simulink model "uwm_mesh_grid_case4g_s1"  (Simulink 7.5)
settings: Solver=ode45  StartTime=0.0  StopTime=8.0  RelTol=1e-4
undefined symbols (not defined in the file or in its folder): D1, Delta, dfilt, DiscIntNeverNeededParam
libraries: powerlib x90, powerlib_extras x24, dsparch4 x6
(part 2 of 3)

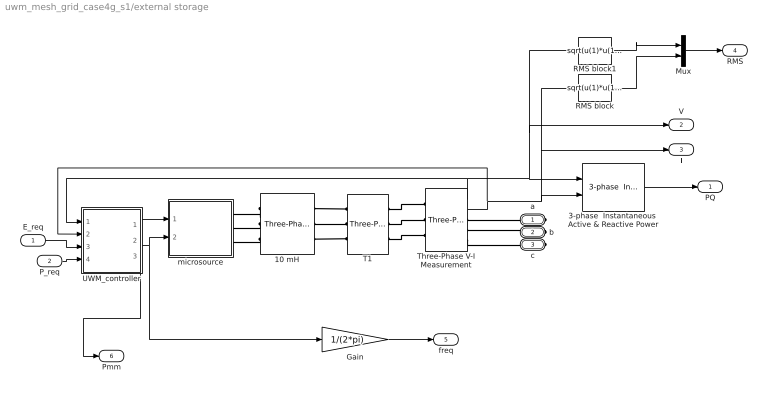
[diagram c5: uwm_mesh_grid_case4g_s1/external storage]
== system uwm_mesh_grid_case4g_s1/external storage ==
  E_req : Inport
  P_req : Inport  Port=2
  10 mH : powerlib/Elements/Three-Phase Series RLC Branch  DialogController=POWERSYS.PowerSysDialog  PhysicalDomain=powersysdomain  SubClassName=unknown  LeftPortType=p1  RightPortType=p1  LConnTagsString=A|B|C  RConnTagsString=A|B|C  BranchType=L  Resistance=.0028  Inductance=5e-3  Capacitance=1e-6  Measurements=None
  3-phase  Instantaneous  Active & Reactive Power : powerlib_extras/Measurements/3-phase  Instantaneous  Active & Reactive Power  DialogController=POWERSYS.PowerSysDialog  SystemSampleTime=-1
  Gain : Gain  Gain=1/(2*pi)  ParameterDataType=fixdt(1, 16)  ParameterScaling=2^0  OutDataType=fixdt(1, 16)  OutScaling=2^0
  Mux : Mux  Inputs=2
  RMS block : Fcn  Expr=sqrt(u(1)*u(1)+u(2)*u(2)+u(3)*u(3))/sqrt(3)
  RMS block1 : Fcn  Expr=sqrt(u(1)*u(1)+u(2)*u(2)+u(3)*u(3))/sqrt(3)
  T1 : powerlib/Elements/Three-Phase Transformer (Two Windings)  DialogController=POWERSYS.PowerSysDialog  SystemSampleTime=-1  Winding1Connection=Delta (D1)  UNITS=SI  NominalPower=[ 45e3 , 60 ]  Winding1=[208 0.02688 0.1075/(2*pi*60)]  Winding2Connection=Yg  Winding2=[208 0.005047 .0201/(2*pi*60)]  SetSaturation=off  Rm=100.e6  Lm=7650.8  Saturation=[0 0;1359.8 0.93633;5.6659e+05 1.186]  Hysteresis=off  DataFile='hysteresis'  SetInitialFlux=off  InitialFluxes=[0.62422 -0.62422 0.54618]  Measurements=None  MoreParameters=off  BreakLoop=off  DataType=on  TransfoNumber=1
  Three-Phase V-I Measurement : powerlib/Measurements/Three-Phase V-I Measurement  DialogController=POWERSYS.PowerSysDialog  SystemSampleTime=-1  VoltageMeasurement=phase-to-ground  SetLabelV=off  LabelV=Vabc  Vpu=off  VpuLL=off  CurrentMeasurement=yes  SetLabelI=off  LabelI=Iabc  Ipu=off  Pbase=100e6  Vbase=500e3  OutputType=Complex  PhasorSimulation=off  PSBequivalent=0
  UWM_controller : Subsystem  mask{Vbase=208, Sbase=15000}
  microsource : Subsystem
  a : PMIOPort  Port=1  Side=Right
  b : PMIOPort  Port=2  Side=Right
  c : PMIOPort  Port=3  Side=Right
  PQ : Outport  OutDataType=fixdt(1, 16)  OutScaling=2^0
  V : Outport  Port=2  OutDataType=fixdt(1, 16)  OutScaling=2^0
  I : Outport  Port=3  OutDataType=fixdt(1, 16)  OutScaling=2^0
  RMS : Outport  Port=4  OutDataType=fixdt(1, 16)  OutScaling=2^0
  freq : Outport  Port=5  OutDataType=fixdt(1, 16)  OutScaling=2^0
  Pmm : Outport  Port=6
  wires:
  E_req/1 -> UWM_controller/3(E_req)
  P_req/1 -> UWM_controller/4(P_req)
  Three-Phase V-I Measurement/1 -> UWM_controller/1(v_meas), 3-phase  Instantaneous  Active & Reactive Power/1, RMS block1/1, V/1
  Three-Phase V-I Measurement/2 -> UWM_controller/2(i_meas), 3-phase  Instantaneous  Active & Reactive Power/2, RMS block/1, I/1
  UWM_controller/1(Vpk) -> microsource/1(Vpk)
  UWM_controller/2(w) -> microsource/2(w), Gain/1
  Gain/1 -> freq/1
  3-phase  Instantaneous  Active & Reactive Power/1 -> PQ/1
  RMS block1/1 -> Mux/1
  RMS block/1 -> Mux/2
  Mux/1 -> RMS/1
  UWM_controller/3(Pmm) -> Pmm/1
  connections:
  b/RConn1 -- Three-Phase V-I Measurement/RConn2
  Three-Phase V-I Measurement/RConn3 -- c/RConn1
  10 mH/LConn2 -- microsource/RConn2
  10 mH/LConn1 -- microsource/RConn1
  10 mH/LConn3 -- microsource/RConn3
  T1/LConn1 -- 10 mH/RConn1
  T1/LConn2 -- 10 mH/RConn2
  T1/LConn3 -- 10 mH/RConn3
  T1/RConn1 -- Three-Phase V-I Measurement/LConn1
  T1/RConn2 -- Three-Phase V-I Measurement/LConn2
  T1/RConn3 -- Three-Phase V-I Measurement/LConn3
  a/RConn1 -- Three-Phase V-I Measurement/RConn1

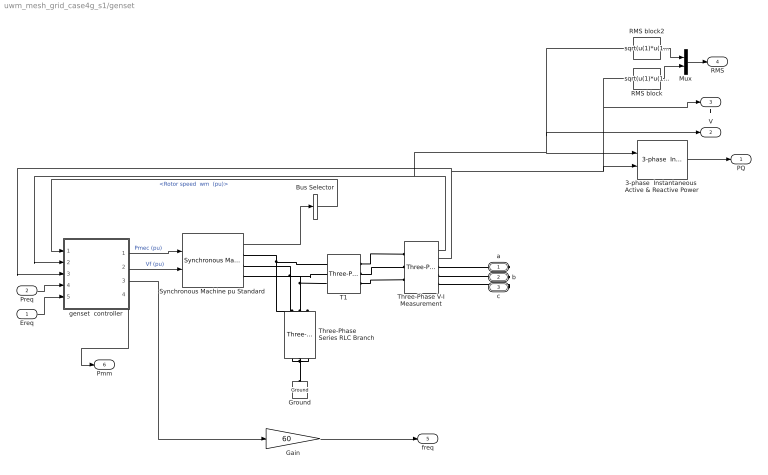
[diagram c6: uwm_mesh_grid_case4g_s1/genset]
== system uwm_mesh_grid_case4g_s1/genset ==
  Ereq : Inport  OutDataType=fixdt(1, 16)  OutScaling=2^0
  Preq : Inport  Port=2  OutDataType=fixdt(1, 16)  OutScaling=2^0
  3-phase  Instantaneous  Active & Reactive Power : powerlib_extras/Measurements/3-phase  Instantaneous  Active & Reactive Power  DialogController=POWERSYS.PowerSysDialog  SystemSampleTime=-1
  Bus Selector : BusSelector  OutputSignals="Mechanical.Rotor speed  wm  (pu)"
  Gain : Gain  Gain=60  ParameterDataType=fixdt(1, 16)  ParameterScaling=2^0  OutDataType=fixdt(1, 16)  OutScaling=2^0
  Ground : powerlib/Elements/Ground  DialogController=POWERSYS.PowerSysDialog  PhysicalDomain=powersysdomain  SubClassName=unknown  LeftPortType=p1  RightPortType=p1  LConnTagsString=a
  Mux : Mux  Inputs=2
  RMS block : Fcn  Expr=sqrt(u(1)*u(1)+u(2)*u(2)+u(3)*u(3))/sqrt(3)
  RMS block2 : Fcn  Expr=sqrt(u(1)*u(1)+u(2)*u(2)+u(3)*u(3))/sqrt(3)
  Synchronous Machine pu Standard : powerlib/Machines/Synchronous Machine pu Standard  DialogController=POWERSYS.PowerSysDialog  SystemSampleTime=-1  PresetModel=No  MechanicalLoad=Mechanical power Pm  ShowDetailedParameters=on  RotorType=Salient-pole  NominalParameters="[ 12500  208   60]"  Reactances1=[ 1.81, 0.3, 0.23, 1.76, 0.65, 0.25, 0.15 ]  Reactances2="[ 1.204, 0.125, 0.056, 0.533,  0.051,  0.037 ]"  dAxisTimeConstants=Short-circuit  qAxisTimeConstants=Short-circuit  TimeConstants1="[ 4.4849  0.0681  0.1  ]"  TimeConstants2=[ 8.0, 0.03, 1.0, 0.07 ]  TimeConstants3="[  .35523  0.00015  0.067  ]"  TimeConstants4=[ 8.0, 0.03, 0.3371, 0.0295 ]  TimeConstants5=[ 1.01, 0.053, 0.1 ]  TimeConstants6=[ 1.3201, 0.023, 1.0, 0.07 ]  TimeConstants7=[0.35523 0.00015 0.0067]  TimeConstants8=[ 1.3201, 0.0231, 0.3371, 0.0295 ]  StatorResistance=0.0217  Mechanical=[ .19 0 2 ]  PolePairs=2  InitialConditions="[ 0  0  0  0  0  0  0  0  1 ]"  SetSaturation=off  Saturation=[0.6404,0.7127,0.8441,0.9214,0.9956,1.082,1.19,1.316,1.457;0.7,0.7698,0.8872,0.9466,0.9969,1.046,1.1,1.151,1.201]  Units=per unit standard parameters  LoadFlowParameters=[1 0 0 0 0]  TsPowergui=0  TsBlock=-1  IterativeModel=Forward Euler
  T1 : powerlib/Elements/Three-Phase Transformer (Two Windings)  DialogController=POWERSYS.PowerSysDialog  SystemSampleTime=-1  Winding1Connection=Delta (D1)  UNITS=SI  NominalPower=[ 45e3 , 60 ]  Winding1=[208 .02688 .10752/(2*pi*60)]  Winding2Connection=Yg  Winding2=[208 .005047 .201899/(2*pi*60)]  SetSaturation=off  Rm=1e+08  Lm=7650.8  Saturation=[0 0;1359.8 0.93633;5.6659e+05 1.186]  Hysteresis=off  DataFile='hysteresis'  SetInitialFlux=off  InitialFluxes=[0.62422 -0.62422 0.54618]  Measurements=None  MoreParameters=off  BreakLoop=off  DataType=on  TransfoNumber=1
  Three-Phase Series RLC Branch : powerlib/Elements/Three-Phase Series RLC Branch  DialogController=POWERSYS.PowerSysDialog  PhysicalDomain=powersysdomain  SubClassName=unknown  LeftPortType=p1  RightPortType=p1  LConnTagsString=A|B|C  RConnTagsString=A|B|C  BranchType=C  Resistance=1  Inductance=1e-3  Capacitance=1.e-4  Measurements=None
  Three-Phase V-I Measurement : powerlib/Measurements/Three-Phase V-I Measurement  DialogController=POWERSYS.PowerSysDialog  SystemSampleTime=-1  VoltageMeasurement=phase-to-ground  SetLabelV=off  LabelV=Vabc  Vpu=off  VpuLL=off  CurrentMeasurement=yes  SetLabelI=off  LabelI=Iabc  Ipu=off  Pbase=100e6  Vbase=500e3  OutputType=Complex  PhasorSimulation=off  PSBequivalent=0
  genset  controller : Subsystem  mask{Vbase=208, Sbase=12500}
  a : PMIOPort  Port=1  Side=Right
  b : PMIOPort  Port=2  Side=Right
  c : PMIOPort  Port=3  Side=Right
  PQ : Outport  OutDataType=fixdt(1, 16)  OutScaling=2^0
  V : Outport  Port=2  OutDataType=fixdt(1, 16)  OutScaling=2^0
  I : Outport  Port=3  OutDataType=fixdt(1, 16)  OutScaling=2^0
  RMS : Outport  Port=4  OutDataType=fixdt(1, 16)  OutScaling=2^0
  freq : Outport  Port=5  OutDataType=fixdt(1, 16)  OutScaling=2^0
  Pmm : Outport  Port=6
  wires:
  genset  controller/1(Pmech) -> Synchronous Machine pu Standard/1  "Pmec (pu)"
  genset  controller/2(Vf) -> Synchronous Machine pu Standard/2  "Vf (pu)"
  Synchronous Machine pu Standard/1 -> Bus Selector/1
  Bus Selector/1 -> genset  controller/1(wr)  "<Rotor speed  wm  (pu)>"
  Three-Phase V-I Measurement/1 -> genset  controller/2(Vabc), 3-phase  Instantaneous  Active & Reactive Power/1, RMS block2/1, V/1
  Three-Phase V-I Measurement/2 -> genset  controller/3(Iabc), 3-phase  Instantaneous  Active & Reactive Power/2, RMS block/1, I/1
  Preq/1 -> genset  controller/4(Preq)
  Ereq/1 -> genset  controller/5(Ereq1)
  genset  controller/3(w) -> Gain/1
  Gain/1 -> freq/1
  3-phase  Instantaneous  Active & Reactive Power/1 -> PQ/1
  RMS block2/1 -> Mux/1
  RMS block/1 -> Mux/2
  Mux/1 -> RMS/1
  genset  controller/4(Pmm) -> Pmm/1
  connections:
  Three-Phase Series RLC Branch/RConn2 -- Three-Phase Series RLC Branch/RConn1 -- Ground/LConn1 -- Three-Phase Series RLC Branch/RConn3
  Synchronous Machine pu Standard/RConn1 -- T1/LConn1 -- Three-Phase Series RLC Branch/LConn1
  Synchronous Machine pu Standard/RConn2 -- T1/LConn2 -- Three-Phase Series RLC Branch/LConn2
  Synchronous Machine pu Standard/RConn3 -- T1/LConn3 -- Three-Phase Series RLC Branch/LConn3
  T1/RConn2 -- Three-Phase V-I Measurement/LConn2
  T1/RConn1 -- Three-Phase V-I Measurement/LConn1
  T1/RConn3 -- Three-Phase V-I Measurement/LConn3
  Three-Phase V-I Measurement/RConn1 -- a/RConn1
  b/RConn1 -- Three-Phase V-I Measurement/RConn2
  c/RConn1 -- Three-Phase V-I Measurement/RConn3

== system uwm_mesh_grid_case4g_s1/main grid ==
  4.16kV 2500kVA : powerlib/Electrical Sources/Three-Phase Source  DialogController=POWERSYS.PowerSysDialog  SystemSampleTime=-1  Voltage=4160  PhaseAngle=0  Frequency=60  InternalConnection=Yg  SpecifyImpedance=on  Resistance=25^2/1000/10  Inductance=25^2/1000/377  ShortCircuitLevel=1200e6  BaseVoltage=4160  XRratio=100
  PC1 : Subsystem  mask{R=.093400, L=.025500, C=2894.3}
  T1 : powerlib/Elements/Three-Phase Transformer (Two Windings)  DialogController=POWERSYS.PowerSysDialog  SystemSampleTime=-1  Winding1Connection=Delta (D1)  UNITS=SI  NominalPower=[ 2500e3 , 60 ]  Winding1=[4160 .04706 .1882/(2*pi*60)]  Winding2Connection=Yg  Winding2=[480 .000627 .0025068/(2*pi*60)]  SetSaturation=off  Rm=1.e6  Lm=1.e6  Saturation=[0 0;589.26 2.1608;2.4552e+05 2.737]  Hysteresis=off  DataFile='hysteresis'  SetInitialFlux=off  InitialFluxes=[1.4405 -1.4405 1.2604]  Measurements=None  MoreParameters=off  BreakLoop=off  DataType=on  TransfoNumber=1
  T2 : powerlib/Elements/Three-Phase Transformer (Two Windings)  DialogController=POWERSYS.PowerSysDialog  SystemSampleTime=-1  Winding1Connection=Delta (D1)  UNITS=SI  NominalPower=[ 75e3 , 60 ]  Winding1=[480 .0169 .0676/(2*pi*60)]  Winding2Connection=Yg  Winding2=[208 .0003 .0127/(2*pi*60)]  SetSaturation=off  Rm=1.e6  Lm=1.e6  Saturation=[0 0;589.26 2.1608;2.4552e+05 2.737]  Hysteresis=off  DataFile='hysteresis'  SetInitialFlux=off  InitialFluxes=[1.4405 -1.4405 1.2604]  Measurements=None  MoreParameters=off  BreakLoop=off  DataType=on  TransfoNumber=1
  A : PMIOPort  Port=1  Side=Right
  B : PMIOPort  Port=2  Side=Right
  C : PMIOPort  Port=3  Side=Right
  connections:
  A/RConn1 -- T2/RConn1
  B/RConn1 -- T2/RConn2
  C/RConn1 -- T2/RConn3
  T1/RConn1 -- PC1/LConn1
  T1/RConn2 -- PC1/LConn2
  T1/RConn3 -- PC1/LConn3
  PC1/RConn1 -- T2/LConn1
  PC1/RConn2 -- T2/LConn2
  PC1/RConn3 -- T2/LConn3
  4.16kV 2500kVA/RConn2 -- T1/LConn2
  4.16kV 2500kVA/RConn1 -- T1/LConn1
  4.16kV 2500kVA/RConn3 -- T1/LConn3

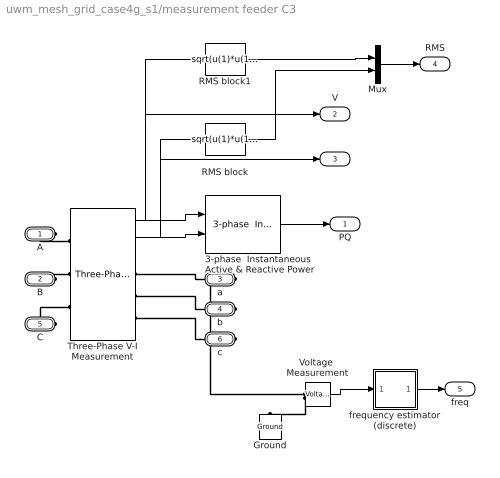
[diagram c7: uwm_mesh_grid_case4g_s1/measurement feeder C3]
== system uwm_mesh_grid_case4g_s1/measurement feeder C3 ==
  3-phase  Instantaneous  Active & Reactive Power : powerlib_extras/Measurements/3-phase  Instantaneous  Active & Reactive Power  DialogController=POWERSYS.PowerSysDialog  SystemSampleTime=-1
  Ground : powerlib/Elements/Ground  DialogController=POWERSYS.PowerSysDialog  PhysicalDomain=powersysdomain  SubClassName=unknown  LeftPortType=p1  RightPortType=p1  LConnTagsString=a
  Mux : Mux  Inputs=2
  RMS block : Fcn  Expr=sqrt(u(1)*u(1)+u(2)*u(2)+u(3)*u(3))/sqrt(3)
  RMS block1 : Fcn  Expr=sqrt(u(1)*u(1)+u(2)*u(2)+u(3)*u(3))/sqrt(3)
  Three-Phase V-I Measurement : powerlib/Measurements/Three-Phase V-I Measurement  DialogController=POWERSYS.PowerSysDialog  SystemSampleTime=-1  VoltageMeasurement=phase-to-ground  SetLabelV=off  LabelV=Vabc  Vpu=off  VpuLL=off  CurrentMeasurement=yes  SetLabelI=off  LabelI=Iabc  Ipu=off  Pbase=100e6  Vbase=500e3  OutputType=Complex  PhasorSimulation=off  PSBequivalent=0
  Voltage  Measurement : powerlib/Measurements/Voltage Measurement  DialogController=POWERSYS.PowerSysDialog  SystemSampleTime=-1  PhasorSimulation=off  OutputType=Complex  PSBequivalent=0
  frequency estimator (discrete) : Subsystem  mask{dt=0.010}
      mask prompts: dt "sample time"
  A : PMIOPort  Port=1  Side=Left
  B : PMIOPort  Port=2  Side=Left
  a : PMIOPort  Port=3  Side=Right
  b : PMIOPort  Port=4  Side=Right
  C : PMIOPort  Port=5  Side=Left
  c : PMIOPort  Port=6  Side=Right
  PQ : Outport  OutDataType=fixdt(1, 16)  OutScaling=2^0
  V : Outport  Port=2  OutDataType=fixdt(1, 16)  OutScaling=2^0
  I : Outport  Port=3  OutDataType=fixdt(1, 16)  OutScaling=2^0
  RMS : Outport  Port=4  OutDataType=fixdt(1, 16)  OutScaling=2^0
  freq : Outport  Port=5  OutDataType=fixdt(1, 16)  OutScaling=2^0
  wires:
  Three-Phase V-I Measurement/1 -> 3-phase  Instantaneous  Active & Reactive Power/1, RMS block1/1, V/1
  Three-Phase V-I Measurement/2 -> 3-phase  Instantaneous  Active & Reactive Power/2, RMS block/1, I/1
  3-phase  Instantaneous  Active & Reactive Power/1 -> PQ/1
  RMS block1/1 -> Mux/1
  RMS block/1 -> Mux/2
  Mux/1 -> RMS/1
  Voltage  Measurement/1 -> frequency estimator (discrete)/1(v)
  frequency estimator (discrete)/1(w) -> freq/1
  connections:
  c/RConn1 -- Three-Phase V-I Measurement/RConn3
  C/RConn1 -- Three-Phase V-I Measurement/LConn3
  b/RConn1 -- Three-Phase V-I Measurement/RConn2
  a/RConn1 -- Three-Phase V-I Measurement/RConn1 -- Voltage  Measurement/LConn1
  B/RConn1 -- Three-Phase V-I Measurement/LConn2
  A/RConn1 -- Three-Phase V-I Measurement/LConn1
  Voltage  Measurement/LConn2 -- Ground/LConn1

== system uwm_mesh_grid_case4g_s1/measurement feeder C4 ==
  3-phase  Instantaneous  Active & Reactive Power : powerlib_extras/Measurements/3-phase  Instantaneous  Active & Reactive Power  DialogController=POWERSYS.PowerSysDialog  SystemSampleTime=-1
  Ground : powerlib/Elements/Ground  DialogController=POWERSYS.PowerSysDialog  PhysicalDomain=powersysdomain  SubClassName=unknown  LeftPortType=p1  RightPortType=p1  LConnTagsString=a
  Mux1 : Mux  Inputs=2
  RMS block : Fcn  Expr=sqrt(u(1)*u(1)+u(2)*u(2)+u(3)*u(3))/sqrt(3)
  RMS block1 : Fcn  Expr=sqrt(u(1)*u(1)+u(2)*u(2)+u(3)*u(3))/sqrt(3)
  Three-Phase V-I Measurement1 : powerlib/Measurements/Three-Phase V-I Measurement  DialogController=POWERSYS.PowerSysDialog  SystemSampleTime=-1  VoltageMeasurement=phase-to-ground  SetLabelV=off  LabelV=Vabc  Vpu=off  VpuLL=off  CurrentMeasurement=yes  SetLabelI=off  LabelI=Iabc  Ipu=off  Pbase=100e6  Vbase=500e3  OutputType=Complex  PhasorSimulation=off  PSBequivalent=0
  Voltage  Measurement : powerlib/Measurements/Voltage Measurement  DialogController=POWERSYS.PowerSysDialog  SystemSampleTime=-1  PhasorSimulation=off  OutputType=Complex  PSBequivalent=0
  frequency estimator (discrete) : Subsystem  mask{dt=0.010}
      mask prompts: dt "sample time"
  A : PMIOPort  Port=1  Side=Left
  B : PMIOPort  Port=2  Side=Left
  a : PMIOPort  Port=3  Side=Right
  b : PMIOPort  Port=4  Side=Right
  C : PMIOPort  Port=5  Side=Left
  c : PMIOPort  Port=6  Side=Right
  PQ : Outport  OutDataType=fixdt(1, 16)  OutScaling=2^0
  V : Outport  Port=2  OutDataType=fixdt(1, 16)  OutScaling=2^0
  I : Outport  Port=3  OutDataType=fixdt(1, 16)  OutScaling=2^0
  RMS : Outport  Port=4  OutDataType=fixdt(1, 16)  OutScaling=2^0
  freq : Outport  Port=5  OutDataType=fixdt(1, 16)  OutScaling=2^0
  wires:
  Three-Phase V-I Measurement1/1 -> 3-phase  Instantaneous  Active & Reactive Power/1, RMS block1/1, V/1
  Three-Phase V-I Measurement1/2 -> 3-phase  Instantaneous  Active & Reactive Power/2, RMS block/1, I/1
  3-phase  Instantaneous  Active & Reactive Power/1 -> PQ/1
  RMS block1/1 -> Mux1/1
  Voltage  Measurement/1 -> frequency estimator (discrete)/1(v)
  frequency estimator (discrete)/1(w) -> freq/1
  RMS block/1 -> Mux1/2
  Mux1/1 -> RMS/1
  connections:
  c/RConn1 -- Three-Phase V-I Measurement1/RConn3
  C/RConn1 -- Three-Phase V-I Measurement1/LConn3
  b/RConn1 -- Three-Phase V-I Measurement1/RConn2
  a/RConn1 -- Three-Phase V-I Measurement1/RConn1 -- Voltage  Measurement/LConn1
  B/RConn1 -- Three-Phase V-I Measurement1/LConn2
  A/RConn1 -- Three-Phase V-I Measurement1/LConn1
  Voltage  Measurement/LConn2 -- Ground/LConn1

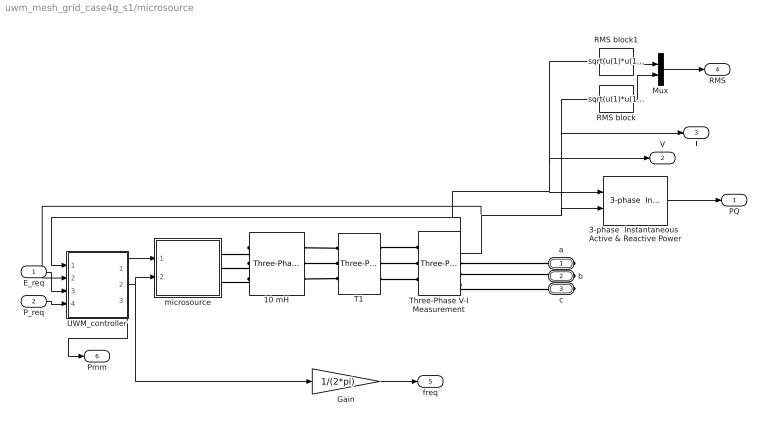
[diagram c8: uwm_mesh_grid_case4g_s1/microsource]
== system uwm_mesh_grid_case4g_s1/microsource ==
  E_req : Inport
  P_req : Inport  Port=2
  10 mH : powerlib/Elements/Three-Phase Series RLC Branch  DialogController=POWERSYS.PowerSysDialog  PhysicalDomain=powersysdomain  SubClassName=unknown  LeftPortType=p1  RightPortType=p1  LConnTagsString=A|B|C  RConnTagsString=A|B|C  BranchType=L  Resistance=.0028  Inductance=5e-3  Capacitance=1e-6  Measurements=None
  3-phase  Instantaneous  Active & Reactive Power : powerlib_extras/Measurements/3-phase  Instantaneous  Active & Reactive Power  DialogController=POWERSYS.PowerSysDialog  SystemSampleTime=-1
  Gain : Gain  Gain=1/(2*pi)  ParameterDataType=fixdt(1, 16)  ParameterScaling=2^0  OutDataType=fixdt(1, 16)  OutScaling=2^0
  Mux : Mux  Inputs=2
  RMS block : Fcn  Expr=sqrt(u(1)*u(1)+u(2)*u(2)+u(3)*u(3))/sqrt(3)
  RMS block1 : Fcn  Expr=sqrt(u(1)*u(1)+u(2)*u(2)+u(3)*u(3))/sqrt(3)
  T1 : powerlib/Elements/Three-Phase Transformer (Two Windings)  DialogController=POWERSYS.PowerSysDialog  SystemSampleTime=-1  Winding1Connection=Delta (D1)  UNITS=SI  NominalPower=[ 45e3 , 60 ]  Winding1=[208 0.02688 0.1075/(2*pi*60)]  Winding2Connection=Yg  Winding2=[208 0.005047 .0201/(2*pi*60)]  SetSaturation=off  Rm=100.e6  Lm=7650.8  Saturation=[0 0;1359.8 0.93633;5.6659e+05 1.186]  Hysteresis=off  DataFile='hysteresis'  SetInitialFlux=off  InitialFluxes=[0.62422 -0.62422 0.54618]  Measurements=None  MoreParameters=off  BreakLoop=off  DataType=on  TransfoNumber=1
  Three-Phase V-I Measurement : powerlib/Measurements/Three-Phase V-I Measurement  DialogController=POWERSYS.PowerSysDialog  SystemSampleTime=-1  VoltageMeasurement=phase-to-ground  SetLabelV=off  LabelV=Vabc  Vpu=off  VpuLL=off  CurrentMeasurement=yes  SetLabelI=off  LabelI=Iabc  Ipu=off  Pbase=100e6  Vbase=500e3  OutputType=Complex  PhasorSimulation=off  PSBequivalent=0
  UWM_controller : Subsystem  mask{Vbase=208, Sbase=15000}
  microsource : Subsystem
  a : PMIOPort  Port=1  Side=Right
  b : PMIOPort  Port=2  Side=Right
  c : PMIOPort  Port=3  Side=Right
  PQ : Outport  OutDataType=fixdt(1, 16)  OutScaling=2^0
  V : Outport  Port=2  OutDataType=fixdt(1, 16)  OutScaling=2^0
  I : Outport  Port=3  OutDataType=fixdt(1, 16)  OutScaling=2^0
  RMS : Outport  Port=4  OutDataType=fixdt(1, 16)  OutScaling=2^0
  freq : Outport  Port=5  OutDataType=fixdt(1, 16)  OutScaling=2^0
  Pmm : Outport  Port=6
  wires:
  E_req/1 -> UWM_controller/3(E_req)
  P_req/1 -> UWM_controller/4(P_req)
  Three-Phase V-I Measurement/1 -> UWM_controller/1(v_meas), 3-phase  Instantaneous  Active & Reactive Power/1, RMS block1/1, V/1
  Three-Phase V-I Measurement/2 -> UWM_controller/2(i_meas), 3-phase  Instantaneous  Active & Reactive Power/2, RMS block/1, I/1
  UWM_controller/1(Vpk) -> microsource/1(Vpk)
  UWM_controller/2(w) -> microsource/2(w), Gain/1
  Gain/1 -> freq/1
  3-phase  Instantaneous  Active & Reactive Power/1 -> PQ/1
  RMS block1/1 -> Mux/1
  RMS block/1 -> Mux/2
  Mux/1 -> RMS/1
  UWM_controller/3(Pmm) -> Pmm/1
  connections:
  b/RConn1 -- Three-Phase V-I Measurement/RConn2
  Three-Phase V-I Measurement/RConn3 -- c/RConn1
  10 mH/LConn2 -- microsource/RConn2
  10 mH/LConn1 -- microsource/RConn1
  10 mH/LConn3 -- microsource/RConn3
  T1/LConn1 -- 10 mH/RConn1
  T1/LConn2 -- 10 mH/RConn2
  T1/LConn3 -- 10 mH/RConn3
  T1/RConn1 -- Three-Phase V-I Measurement/LConn1
  T1/RConn2 -- Three-Phase V-I Measurement/LConn2
  T1/RConn3 -- Three-Phase V-I Measurement/LConn3
  a/RConn1 -- Three-Phase V-I Measurement/RConn1

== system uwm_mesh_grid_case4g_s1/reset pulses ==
  Sum : Sum  Inputs=|++  OutDataType=fixdt(1, 16)  OutScaling=2^0
  pulse : Subsystem  mask{tstart=tpulse(1), dt=.1}
  pulse1 : Subsystem  mask{tstart=tpulse(2), dt=.1}
  Out1 : Outport
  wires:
  pulse/1(Out1) -> Sum/1
  pulse1/1(Out1) -> Sum/2
  Sum/1 -> Out1/1

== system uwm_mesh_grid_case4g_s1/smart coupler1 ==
  event : Inport  OutDataType=fixdt(1, 16)  OutScaling=2^0
  Abs : Abs  OutDataType=fixdt(1, 16)  OutScaling=2^0
  Level-2 M-file S-Function : M-S-Function  FunctionName=smart_coupler
  SS2 : powerlib/Elements/Three-Phase Breaker  DialogController=POWERSYS.PowerSysDialog  SystemSampleTime=-1  InitialState=open  SwitchA=on  SwitchB=on  SwitchC=on  SwitchTimes=[5 6]  External=on  BreakerResistance=.001  SnubberResistance=1e6  SnubberCapacitance=inf  Measurements=None
  Scope : Scope  NumInputPorts=3
  Transfer Fcn : TransferFcn  Numerator=[100]  Denominator=[1 100]
  Voltage Measurement : powerlib/Measurements/Voltage Measurement  DialogController=POWERSYS.PowerSysDialog  SystemSampleTime=-1  PhasorSimulation=off  OutputType=Complex  PSBequivalent=0
  A : PMIOPort  Port=1  Side=Left
  B : PMIOPort  Port=2  Side=Left
  C : PMIOPort  Port=3  Side=Left
  a : PMIOPort  Port=4  Side=Right
  b : PMIOPort  Port=5  Side=Right
  c : PMIOPort  Port=6  Side=Right
  connected : Outport  OutDataType=fixdt(1, 16)  OutScaling=2^0
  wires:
  Level-2 M-file S-Function/1 -> Scope/1, SS2/1, connected/1
  Voltage Measurement/1 -> Abs/1
  Abs/1 -> Transfer Fcn/1
  Transfer Fcn/1 -> Level-2 M-file S-Function/1, Scope/3
  event/1 -> Level-2 M-file S-Function/2, Scope/2
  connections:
  A/RConn1 -- SS2/LConn1 -- Voltage Measurement/LConn1
  Voltage Measurement/LConn2 -- a/RConn1 -- SS2/RConn1
  B/RConn1 -- SS2/LConn2
  C/RConn1 -- SS2/LConn3
  b/RConn1 -- SS2/RConn2
  c/RConn1 -- SS2/RConn3

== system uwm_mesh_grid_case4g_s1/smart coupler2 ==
  event : Inport  OutDataType=fixdt(1, 16)  OutScaling=2^0
  Abs : Abs  OutDataType=fixdt(1, 16)  OutScaling=2^0
  Level-2 M-file S-Function : M-S-Function  FunctionName=smart_coupler
  SS2 : powerlib/Elements/Three-Phase Breaker  DialogController=POWERSYS.PowerSysDialog  SystemSampleTime=-1  InitialState=open  SwitchA=on  SwitchB=on  SwitchC=on  SwitchTimes=[5 6]  External=on  BreakerResistance=.001  SnubberResistance=1e6  SnubberCapacitance=inf  Measurements=None
  Scope : Scope  NumInputPorts=3
  Transfer Fcn : TransferFcn  Numerator=[100]  Denominator=[1 100]
  Voltage Measurement : powerlib/Measurements/Voltage Measurement  DialogController=POWERSYS.PowerSysDialog  SystemSampleTime=-1  PhasorSimulation=off  OutputType=Complex  PSBequivalent=0
  A : PMIOPort  Port=1  Side=Left
  B : PMIOPort  Port=2  Side=Left
  C : PMIOPort  Port=3  Side=Left
  a : PMIOPort  Port=4  Side=Right
  b : PMIOPort  Port=5  Side=Right
  c : PMIOPort  Port=6  Side=Right
  connected : Outport  OutDataType=fixdt(1, 16)  OutScaling=2^0
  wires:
  Level-2 M-file S-Function/1 -> Scope/1, SS2/1, connected/1
  Voltage Measurement/1 -> Abs/1
  Abs/1 -> Transfer Fcn/1
  Transfer Fcn/1 -> Level-2 M-file S-Function/1, Scope/3
  event/1 -> Level-2 M-file S-Function/2, Scope/2
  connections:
  A/RConn1 -- SS2/LConn1 -- Voltage Measurement/LConn1
  Voltage Measurement/LConn2 -- a/RConn1 -- SS2/RConn1
  B/RConn1 -- SS2/LConn2
  C/RConn1 -- SS2/LConn3
  b/RConn1 -- SS2/RConn2
  c/RConn1 -- SS2/RConn3

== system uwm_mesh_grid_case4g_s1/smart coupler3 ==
  event : Inport  OutDataType=fixdt(1, 16)  OutScaling=2^0
  Abs : Abs  OutDataType=fixdt(1, 16)  OutScaling=2^0
  Level-2 M-file S-Function : M-S-Function  FunctionName=smart_coupler
  SS2 : powerlib/Elements/Three-Phase Breaker  DialogController=POWERSYS.PowerSysDialog  SystemSampleTime=-1  InitialState=open  SwitchA=on  SwitchB=on  SwitchC=on  SwitchTimes=[5 6]  External=on  BreakerResistance=.001  SnubberResistance=1e6  SnubberCapacitance=inf  Measurements=None
  Scope : Scope  NumInputPorts=3
  Transfer Fcn : TransferFcn  Numerator=[100]  Denominator=[1 100]
  Voltage Measurement : powerlib/Measurements/Voltage Measurement  DialogController=POWERSYS.PowerSysDialog  SystemSampleTime=-1  PhasorSimulation=off  OutputType=Complex  PSBequivalent=0
  A : PMIOPort  Port=1  Side=Left
  B : PMIOPort  Port=2  Side=Left
  C : PMIOPort  Port=3  Side=Left
  a : PMIOPort  Port=4  Side=Right
  b : PMIOPort  Port=5  Side=Right
  c : PMIOPort  Port=6  Side=Right
  connected : Outport  OutDataType=fixdt(1, 16)  OutScaling=2^0
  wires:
  Level-2 M-file S-Function/1 -> Scope/1, SS2/1, connected/1
  Voltage Measurement/1 -> Abs/1
  Abs/1 -> Transfer Fcn/1
  Transfer Fcn/1 -> Level-2 M-file S-Function/1, Scope/3
  event/1 -> Level-2 M-file S-Function/2, Scope/2
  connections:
  A/RConn1 -- SS2/LConn1 -- Voltage Measurement/LConn1
  Voltage Measurement/LConn2 -- a/RConn1 -- SS2/RConn1
  B/RConn1 -- SS2/LConn2
  C/RConn1 -- SS2/LConn3
  b/RConn1 -- SS2/RConn2
  c/RConn1 -- SS2/RConn3

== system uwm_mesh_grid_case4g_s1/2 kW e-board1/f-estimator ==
  v : Inport
  Constant : Constant  Value=60  OutDataType=fixdt(1, 16)  OutScaling=2^0
  Fcn : Fcn  Expr=sin(2*pi*u[1])
  Filter1 : dsparch4/Biquad Filter  Tag=BlockMethodSubSystem  DialogController=dspdialog.BiquadFilter  DialogControllerArgs=DataTag0  IIRFiltStruct=Direct form II  CoeffSource=Specify via dialog  BiQuadCoeffs=[1 -1.36 1 1 -1.78 0.87;1 1 0 1 -0.85 0]  a0Flag=Warning  IC=0  ICnum=0  ICden=0  denAccumFracLength=30  denProdOutputFracLength=30  secondMemoryFracLength=15  roundingMode=Floor  overflowMode=off  ScaleValues=[0.05;0.23;1]  optimizeScaleValues=on  ScaleValueMode=Specify via input port (g)  scaleValueFracLength=14  FilterSource=Specify via dialog  dfiltObjectName=dfilt.df2tsos([1 0.3 0.4],[1 0.1 0.2])
  Gain : Gain  Gain=1/150  ParameterDataType=fixdt(1, 16)  ParameterScaling=2^0  OutDataType=fixdt(1, 16)  OutScaling=2^0  SampleTime=dt
  Product : Product  OutDataType=fixdt(1, 16)  OutScaling=2^0
  Scope : Scope
  Sum : Sum  Inputs=|++  OutDataType=fixdt(1, 16)  OutScaling=2^0
  modulo discrete integrator : Subsystem  mask{dt=dt}
      mask prompts: dt "sample time"
  w : Outport  OutDataType=fixdt(1, 16)  OutScaling=2^0
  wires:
  Gain/1 -> Product/1
  v/1 -> Gain/1
  Filter1/1 -> Sum/1, Scope/1
  Product/1 -> Filter1/1
  Sum/1 -> w/1, modulo discrete integrator/1(In1)
  modulo discrete integrator/1(Out1) -> Fcn/1
  Constant/1 -> Sum/2
  Fcn/1 -> Product/2

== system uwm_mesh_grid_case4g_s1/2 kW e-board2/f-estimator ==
  v : Inport
  Constant : Constant  Value=60  OutDataType=fixdt(1, 16)  OutScaling=2^0
  Fcn : Fcn  Expr=sin(2*pi*u[1])
  Filter1 : dsparch4/Biquad Filter  Tag=BlockMethodSubSystem  DialogController=dspdialog.BiquadFilter  DialogControllerArgs=DataTag1  IIRFiltStruct=Direct form II  CoeffSource=Specify via dialog  BiQuadCoeffs=[1 -1.36 1 1 -1.78 0.87;1 1 0 1 -0.85 0]  a0Flag=Warning  IC=0  ICnum=0  ICden=0  denAccumFracLength=30  denProdOutputFracLength=30  secondMemoryFracLength=15  roundingMode=Floor  overflowMode=off  ScaleValues=[0.05;0.23;1]  optimizeScaleValues=on  ScaleValueMode=Specify via input port (g)  scaleValueFracLength=14  FilterSource=Specify via dialog  dfiltObjectName=dfilt.df2tsos([1 0.3 0.4],[1 0.1 0.2])
  Gain : Gain  Gain=1/150  ParameterDataType=fixdt(1, 16)  ParameterScaling=2^0  OutDataType=fixdt(1, 16)  OutScaling=2^0  SampleTime=dt
  Product : Product  OutDataType=fixdt(1, 16)  OutScaling=2^0
  Scope : Scope
  Sum : Sum  Inputs=|++  OutDataType=fixdt(1, 16)  OutScaling=2^0
  modulo discrete integrator : Subsystem  mask{dt=dt}
      mask prompts: dt "sample time"
  w : Outport  OutDataType=fixdt(1, 16)  OutScaling=2^0
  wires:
  Gain/1 -> Product/1
  v/1 -> Gain/1
  Filter1/1 -> Sum/1, Scope/1
  Product/1 -> Filter1/1
  Sum/1 -> w/1, modulo discrete integrator/1(In1)
  modulo discrete integrator/1(Out1) -> Fcn/1
  Constant/1 -> Sum/2
  Fcn/1 -> Product/2

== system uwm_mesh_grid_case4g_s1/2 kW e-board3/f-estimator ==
  v : Inport
  Constant : Constant  Value=60  OutDataType=fixdt(1, 16)  OutScaling=2^0
  Fcn : Fcn  Expr=sin(2*pi*u[1])
  Filter1 : dsparch4/Biquad Filter  Tag=BlockMethodSubSystem  DialogController=dspdialog.BiquadFilter  DialogControllerArgs=DataTag2  IIRFiltStruct=Direct form II  CoeffSource=Specify via dialog  BiQuadCoeffs=[1 -1.36 1 1 -1.78 0.87;1 1 0 1 -0.85 0]  a0Flag=Warning  IC=0  ICnum=0  ICden=0  denAccumFracLength=30  denProdOutputFracLength=30  secondMemoryFracLength=15  roundingMode=Floor  overflowMode=off  ScaleValues=[0.05;0.23;1]  optimizeScaleValues=on  ScaleValueMode=Specify via input port (g)  scaleValueFracLength=14  FilterSource=Specify via dialog  dfiltObjectName=dfilt.df2tsos([1 0.3 0.4],[1 0.1 0.2])
  Gain : Gain  Gain=1/150  ParameterDataType=fixdt(1, 16)  ParameterScaling=2^0  OutDataType=fixdt(1, 16)  OutScaling=2^0  SampleTime=dt
  Product : Product  OutDataType=fixdt(1, 16)  OutScaling=2^0
  Scope : Scope
  Sum : Sum  Inputs=|++  OutDataType=fixdt(1, 16)  OutScaling=2^0
  modulo discrete integrator : Subsystem  mask{dt=dt}
      mask prompts: dt "sample time"
  w : Outport  OutDataType=fixdt(1, 16)  OutScaling=2^0
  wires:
  Gain/1 -> Product/1
  v/1 -> Gain/1
  Filter1/1 -> Sum/1, Scope/1
  Product/1 -> Filter1/1
  Sum/1 -> w/1, modulo discrete integrator/1(In1)
  modulo discrete integrator/1(Out1) -> Fcn/1
  Constant/1 -> Sum/2
  Fcn/1 -> Product/2

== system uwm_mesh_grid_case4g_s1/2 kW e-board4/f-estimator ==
  v : Inport
  Constant : Constant  Value=60  OutDataType=fixdt(1, 16)  OutScaling=2^0
  Fcn : Fcn  Expr=sin(2*pi*u[1])
  Filter1 : dsparch4/Biquad Filter  Tag=BlockMethodSubSystem  DialogController=dspdialog.BiquadFilter  DialogControllerArgs=DataTag3  IIRFiltStruct=Direct form II  CoeffSource=Specify via dialog  BiQuadCoeffs=[1 -1.36 1 1 -1.78 0.87;1 1 0 1 -0.85 0]  a0Flag=Warning  IC=0  ICnum=0  ICden=0  denAccumFracLength=30  denProdOutputFracLength=30  secondMemoryFracLength=15  roundingMode=Floor  overflowMode=off  ScaleValues=[0.05;0.23;1]  optimizeScaleValues=on  ScaleValueMode=Specify via input port (g)  scaleValueFracLength=14  FilterSource=Specify via dialog  dfiltObjectName=dfilt.df2tsos([1 0.3 0.4],[1 0.1 0.2])
  Gain : Gain  Gain=1/150  ParameterDataType=fixdt(1, 16)  ParameterScaling=2^0  OutDataType=fixdt(1, 16)  OutScaling=2^0  SampleTime=dt
  Product : Product  OutDataType=fixdt(1, 16)  OutScaling=2^0
  Scope : Scope
  Sum : Sum  Inputs=|++  OutDataType=fixdt(1, 16)  OutScaling=2^0
  modulo discrete integrator : Subsystem  mask{dt=dt}
      mask prompts: dt "sample time"
  w : Outport  OutDataType=fixdt(1, 16)  OutScaling=2^0
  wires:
  Gain/1 -> Product/1
  v/1 -> Gain/1
  Filter1/1 -> Sum/1, Scope/1
  Product/1 -> Filter1/1
  Sum/1 -> w/1, modulo discrete integrator/1(In1)
  modulo discrete integrator/1(Out1) -> Fcn/1
  Constant/1 -> Sum/2
  Fcn/1 -> Product/2

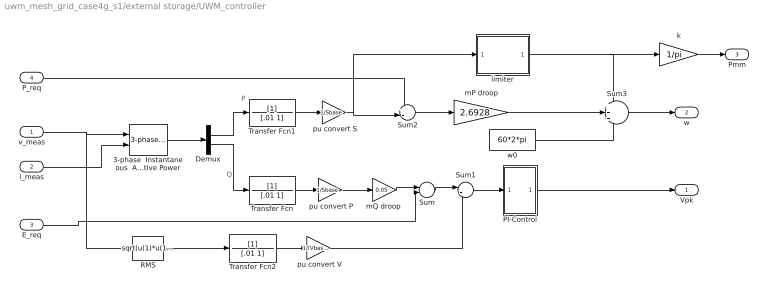
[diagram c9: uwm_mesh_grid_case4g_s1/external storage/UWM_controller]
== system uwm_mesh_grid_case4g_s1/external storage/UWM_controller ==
  note: P
  note: Q
  v_meas : Inport
  i_meas : Inport  Port=2
  E_req : Inport  Port=3
  P_req : Inport  Port=4
  " pu convert P" : Gain  Gain=1/Sbase  ParameterDataType=sfix(16)  ParameterScaling=2^0  OutDataType=sfix(16)  OutScaling=2^0
  " pu convert S" : Gain  Gain=1/Sbase  ParameterDataType=sfix(16)  ParameterScaling=2^0  OutDataType=sfix(16)  OutScaling=2^0
  " pu convert V" : Gain  Gain=1/(Vbase/sqrt(3))  ParameterDataType=sfix(16)  ParameterScaling=2^0  OutDataType=sfix(16)  OutScaling=2^0
  3-phase  Instantaneous  Active & Reactive Power : powerlib_extras/Measurements/3-phase  Instantaneous  Active & Reactive Power  DialogController=POWERSYS.PowerSysDialog  SystemSampleTime=-1
  Demux : Demux  Outputs=2
  PI-Control : Subsystem
  RMS : Fcn  Expr=sqrt(u(1)*u(1)+u(2)*u(2)+u(3)*u(3))/sqrt(3)
  Sum : Sum  Inputs=|-+  OutDataType=sfix(16)  OutScaling=2^0
  Sum1 : Sum  Inputs=|+-  OutDataType=sfix(16)  OutScaling=2^0
  Sum2 : Sum  Inputs=+-|  OutDataType=sfix(16)  OutScaling=2^0
  Sum3 : Sum  Inputs=+++  OutDataType=sfix(16)  OutScaling=2^0
  Transfer Fcn : TransferFcn  Denominator=[.01 1]
  Transfer Fcn1 : TransferFcn  Denominator=[.01 1]
  Transfer Fcn2 : TransferFcn  Denominator=[.01 1]
  k : Gain  Gain=1/pi  ParameterDataType=sfix(16)  ParameterScaling=2^0  OutDataType=sfix(16)  OutScaling=2^0
  limiter : Subsystem
  mP droop : Gain  Gain=2.6928  ParameterDataType=sfix(16)  ParameterScaling=2^0  OutDataType=sfix(16)  OutScaling=2^0
  "mQ droop " : Gain  Gain=0.05  ParameterDataType=sfix(16)  ParameterScaling=2^0  OutDataType=sfix(16)  OutScaling=2^0
  w0 : Constant  Value=60*2*pi  OutDataType=fixdt(1, 16)  OutScaling=2^0
  Vpk : Outport
  w : Outport  Port=2
  Pmm : Outport  Port=3
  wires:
  Transfer Fcn2/1 -> " pu convert V"/1
  Transfer Fcn/1 -> " pu convert P"/1
  " pu convert P"/1 -> "mQ droop "/1
  Transfer Fcn1/1 -> " pu convert S"/1
  " pu convert S"/1 -> limiter/1(In1), Sum2/2
  i_meas/1 -> 3-phase  Instantaneous  Active & Reactive Power/2
  P_req/1 -> Sum2/1
  mP droop/1 -> Sum3/2
  limiter/1(Out1) -> Sum3/1, k/1
  w0/1 -> Sum3/3
  Sum2/1 -> mP droop/1
  Sum1/1 -> PI-Control/1(In1)
  Sum/1 -> Sum1/1
  "mQ droop "/1 -> Sum/1
  RMS/1 -> Transfer Fcn2/1
  Demux/2 -> Transfer Fcn/1
  Demux/1 -> Transfer Fcn1/1
  3-phase  Instantaneous  Active & Reactive Power/1 -> Demux/1
  v_meas/1 -> RMS/1, 3-phase  Instantaneous  Active & Reactive Power/1
  PI-Control/1(Out1) -> Vpk/1
  Sum3/1 -> w/1
  E_req/1 -> Sum/2
  " pu convert V"/1 -> Sum1/2
  k/1 -> Pmm/1

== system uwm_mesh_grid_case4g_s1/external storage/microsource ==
  Vpk : Inport  OutDataType=fixdt(1, 16)  OutScaling=2^0
  w : Inport  Port=2  OutDataType=fixdt(1, 16)  OutScaling=2^0
  Demux : Demux  Outputs=3
  Ground2 : powerlib/Elements/Ground  DialogController=POWERSYS.PowerSysDialog  PhysicalDomain=powersysdomain  SubClassName=unknown  LeftPortType=p1  RightPortType=p1  LConnTagsString=a
  Integrator : Integrator
  Mux : Mux  Inputs=3
  Product : Product  OutDataType=sfix(16)  OutScaling=2^0
  Series RLC Branch : powerlib/Elements/Series RLC Branch  DialogController=POWERSYS.PowerSysDialog  PhysicalDomain=powersysdomain  SubClassName=unknown  LeftPortType=p1  RightPortType=p1  LConnTagsString=__new0  RConnTagsString=__new0  BranchType=C  Resistance=1  Inductance=1e-3  SetiL0=off  InitialCurrent=0  Capacitance=1e-8  Setx0=off  InitialVoltage=0  Measurements=None
  phaseA : powerlib/Electrical Sources/Controlled Voltage Source  DialogController=POWERSYS.PowerSysDialog  SystemSampleTime=-1  Initialize=on  Source_Type=AC  Amplitude=0  Phase=0  Frequency=0  Measurements=None
  phaseB : powerlib/Electrical Sources/Controlled Voltage Source  DialogController=POWERSYS.PowerSysDialog  SystemSampleTime=-1  Initialize=on  Source_Type=AC  Amplitude=0  Phase=0  Frequency=0  Measurements=None
  phaseC : powerlib/Electrical Sources/Controlled Voltage Source  DialogController=POWERSYS.PowerSysDialog  SystemSampleTime=-1  Initialize=on  Source_Type=AC  Amplitude=0  Phase=0  Frequency=0  Measurements=None
  v_A : Fcn  Expr=cos(u)
  v_B : Fcn  Expr=cos(u-2*pi/3)
  v_C : Fcn  Expr=cos(u+2*pi/3)
  Va : PMIOPort  Tag=PMCPort  Port=1  Side=Right
  Vb : PMIOPort  Tag=PMCPort  Port=2  Side=Right
  Vc : PMIOPort  Tag=PMCPort  Port=3  Side=Right
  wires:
  Product/1 -> Demux/1
  Vpk/1 -> Product/1
  Mux/1 -> Product/2
  w/1 -> Integrator/1
  Integrator/1 -> v_A/1, v_B/1, v_C/1
  v_A/1 -> Mux/1
  v_B/1 -> Mux/2
  v_C/1 -> Mux/3
  Demux/1 -> phaseA/1
  Demux/2 -> phaseB/1
  Demux/3 -> phaseC/1
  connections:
  Vb/RConn1 -- phaseB/RConn1 -- phaseA/LConn1
  Va/RConn1 -- phaseC/LConn1 -- phaseA/RConn1
  Vc/RConn1 -- phaseC/RConn1
  Series RLC Branch/LConn1 -- phaseB/LConn1
  Series RLC Branch/RConn1 -- Ground2/LConn1

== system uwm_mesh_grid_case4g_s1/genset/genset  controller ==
  wr : Inport
  Vabc : Inport  Port=2
  Iabc : Inport  Port=3
  Preq : Inport  Port=4
  Ereq1 : Inport  Port=5
  Gain : Gain  ParameterDataType=fixdt(1, 16)  ParameterScaling=2^0  OutDataType=fixdt(1, 16)  OutScaling=2^0
  P-w droop : Subsystem
  PVQ computation : Subsystem
  Q-E droop : Subsystem
  exciter : Subsystem
  ic_engine gpvernor : Subsystem
  Pmech : Outport
  Vf : Outport  Port=2
  w : Outport  Port=3
  Pmm : Outport  Port=4
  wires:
  P-w droop/1(w) -> w/1, ic_engine gpvernor/3(w)
  PVQ computation/1(P_pu) -> P-w droop/2(P), ic_engine gpvernor/2(Pmeas)
  PVQ computation/3(Q_pu) -> Q-E droop/2(Q)
  Q-E droop/1(Vpk) -> exciter/2(Ef_mcd_wr)
  ic_engine gpvernor/1(Pmech) -> Pmech/1
  Vabc/1 -> PVQ computation/1(Vabc)
  Iabc/1 -> PVQ computation/2(Iabc)
  exciter/1(Ef) -> Vf/1
  Preq/1 -> P-w droop/1(P_req)
  Ereq1/1 -> Q-E droop/3(E_req)
  PVQ computation/2(Vt) -> Q-E droop/1(v_meas)
  Gain/1 -> ic_engine gpvernor/1(wr), exciter/1(wr)
  wr/1 -> Gain/1
  P-w droop/2(Pmm) -> Pmm/1

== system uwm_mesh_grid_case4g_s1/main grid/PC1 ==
  Three-Phase Series RLC Branch3 : powerlib/Elements/Three-Phase Series RLC Branch  DialogController=POWERSYS.PowerSysDialog  PhysicalDomain=powersysdomain  SubClassName=unknown  LeftPortType=p1  RightPortType=p1  LConnTagsString=A|B|C  RConnTagsString=A|B|C  BranchType=RL  Resistance=R  Inductance=L  Capacitance=1/(336*2*pi*60)  Measurements=None
  A* : PMIOPort  Tag=PMCPort  Port=1  Side=Right
  B* : PMIOPort  Tag=PMCPort  Port=2  Side=Right
  C* : PMIOPort  Tag=PMCPort  Port=3  Side=Right
  A : PMIOPort  Tag=PMCPort  Port=4  Side=Left
  B : PMIOPort  Tag=PMCPort  Port=5  Side=Left
  C : PMIOPort  Tag=PMCPort  Port=6  Side=Left
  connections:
  A*/RConn1 -- Three-Phase Series RLC Branch3/LConn1
  B*/RConn1 -- Three-Phase Series RLC Branch3/LConn2
  C*/RConn1 -- Three-Phase Series RLC Branch3/LConn3
  Three-Phase Series RLC Branch3/RConn1 -- A/RConn1
  Three-Phase Series RLC Branch3/RConn2 -- B/RConn1
  Three-Phase Series RLC Branch3/RConn3 -- C/RConn1

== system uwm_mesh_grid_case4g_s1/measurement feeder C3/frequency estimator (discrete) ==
  v : Inport
  Constant : Constant  Value=60  OutDataType=fixdt(1, 16)  OutScaling=2^0
  Fcn : Fcn  Expr=sin(2*pi*u[1])
  Filter1 : dsparch4/Biquad Filter  Tag=BlockMethodSubSystem  DialogController=dspdialog.BiquadFilter  DialogControllerArgs=DataTag4  IIRFiltStruct=Direct form II  CoeffSource=Specify via dialog  BiQuadCoeffs=[1 -1.36 1 1 -1.78 0.87;1 1 0 1 -0.85 0]  a0Flag=Warning  IC=0  ICnum=0  ICden=0  denAccumFracLength=30  denProdOutputFracLength=30  secondMemoryFracLength=15  roundingMode=Floor  overflowMode=off  ScaleValues=[0.05;0.23;1]  optimizeScaleValues=on  ScaleValueMode=Specify via input port (g)  scaleValueFracLength=14  FilterSource=Specify via dialog  dfiltObjectName=dfilt.df2tsos([1 0.3 0.4],[1 0.1 0.2])
  Gain : Gain  Gain=1/150  ParameterDataType=fixdt(1, 16)  ParameterScaling=2^0  OutDataType=fixdt(1, 16)  OutScaling=2^0  SampleTime=dt
  Product : Product  OutDataType=fixdt(1, 16)  OutScaling=2^0
  Scope : Scope
  Sum : Sum  Inputs=|++  OutDataType=fixdt(1, 16)  OutScaling=2^0
  modulo discrete integrator : Subsystem  mask{dt=dt}
      mask prompts: dt "sample time"
  w : Outport  OutDataType=fixdt(1, 16)  OutScaling=2^0
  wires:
  Fcn/1 -> Product/2
  Constant/1 -> Sum/2
  modulo discrete integrator/1(Out1) -> Fcn/1
  Sum/1 -> modulo discrete integrator/1(In1), w/1
  Product/1 -> Filter1/1
  Filter1/1 -> Scope/1, Sum/1
  v/1 -> Gain/1
  Gain/1 -> Product/1

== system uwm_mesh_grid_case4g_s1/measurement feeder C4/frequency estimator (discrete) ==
  v : Inport
  Constant : Constant  Value=60  OutDataType=fixdt(1, 16)  OutScaling=2^0
  Fcn : Fcn  Expr=sin(2*pi*u[1])
  Filter1 : dsparch4/Biquad Filter  Tag=BlockMethodSubSystem  DialogController=dspdialog.BiquadFilter  DialogControllerArgs=DataTag5  IIRFiltStruct=Direct form II  CoeffSource=Specify via dialog  BiQuadCoeffs=[1 -1.36 1 1 -1.78 0.87;1 1 0 1 -0.85 0]  a0Flag=Warning  IC=0  ICnum=0  ICden=0  denAccumFracLength=30  denProdOutputFracLength=30  secondMemoryFracLength=15  roundingMode=Floor  overflowMode=off  ScaleValues=[0.05;0.23;1]  optimizeScaleValues=on  ScaleValueMode=Specify via input port (g)  scaleValueFracLength=14  FilterSource=Specify via dialog  dfiltObjectName=dfilt.df2tsos([1 0.3 0.4],[1 0.1 0.2])
  Gain : Gain  Gain=1/150  ParameterDataType=fixdt(1, 16)  ParameterScaling=2^0  OutDataType=fixdt(1, 16)  OutScaling=2^0  SampleTime=dt
  Product : Product  OutDataType=fixdt(1, 16)  OutScaling=2^0
  Scope : Scope
  Sum : Sum  Inputs=|++  OutDataType=fixdt(1, 16)  OutScaling=2^0
  modulo discrete integrator : Subsystem  mask{dt=dt}
      mask prompts: dt "sample time"
  w : Outport  OutDataType=fixdt(1, 16)  OutScaling=2^0
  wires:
  Fcn/1 -> Product/2
  Constant/1 -> Sum/2
  modulo discrete integrator/1(Out1) -> Fcn/1
  Sum/1 -> modulo discrete integrator/1(In1), w/1
  Product/1 -> Filter1/1
  Filter1/1 -> Scope/1, Sum/1
  v/1 -> Gain/1
  Gain/1 -> Product/1

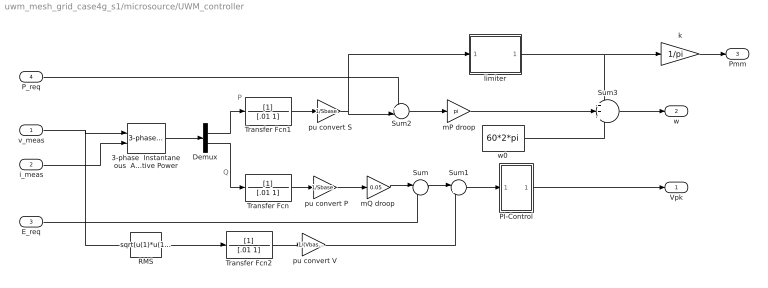
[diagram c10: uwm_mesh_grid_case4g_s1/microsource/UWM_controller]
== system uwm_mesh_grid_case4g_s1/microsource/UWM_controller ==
  note: P
  note: Q
  v_meas : Inport
  i_meas : Inport  Port=2
  E_req : Inport  Port=3
  P_req : Inport  Port=4
  " pu convert P" : Gain  Gain=1/Sbase  ParameterDataType=sfix(16)  ParameterScaling=2^0  OutDataType=sfix(16)  OutScaling=2^0
  " pu convert S" : Gain  Gain=1/Sbase  ParameterDataType=sfix(16)  ParameterScaling=2^0  OutDataType=sfix(16)  OutScaling=2^0
  " pu convert V" : Gain  Gain=1/(Vbase/sqrt(3))  ParameterDataType=sfix(16)  ParameterScaling=2^0  OutDataType=sfix(16)  OutScaling=2^0
  3-phase  Instantaneous  Active & Reactive Power : powerlib_extras/Measurements/3-phase  Instantaneous  Active & Reactive Power  DialogController=POWERSYS.PowerSysDialog  SystemSampleTime=-1
  Demux : Demux  Outputs=2
  PI-Control : Subsystem
  RMS : Fcn  Expr=sqrt(u(1)*u(1)+u(2)*u(2)+u(3)*u(3))/sqrt(3)
  Sum : Sum  Inputs=|-+  OutDataType=sfix(16)  OutScaling=2^0
  Sum1 : Sum  Inputs=|+-  OutDataType=sfix(16)  OutScaling=2^0
  Sum2 : Sum  Inputs=+-|  OutDataType=sfix(16)  OutScaling=2^0
  Sum3 : Sum  Inputs=+++  OutDataType=sfix(16)  OutScaling=2^0
  Transfer Fcn : TransferFcn  Denominator=[.01 1]
  Transfer Fcn1 : TransferFcn  Denominator=[.01 1]
  Transfer Fcn2 : TransferFcn  Denominator=[.01 1]
  k : Gain  Gain=1/pi  ParameterDataType=sfix(16)  ParameterScaling=2^0  OutDataType=sfix(16)  OutScaling=2^0
  limiter : Subsystem
  mP droop : Gain  Gain=pi  ParameterDataType=sfix(16)  ParameterScaling=2^0  OutDataType=sfix(16)  OutScaling=2^0
  "mQ droop " : Gain  Gain=0.05  ParameterDataType=sfix(16)  ParameterScaling=2^0  OutDataType=sfix(16)  OutScaling=2^0
  w0 : Constant  Value=60*2*pi  OutDataType=fixdt(1, 16)  OutScaling=2^0
  Vpk : Outport
  w : Outport  Port=2
  Pmm : Outport  Port=3
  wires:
  Transfer Fcn2/1 -> " pu convert V"/1
  Transfer Fcn/1 -> " pu convert P"/1
  " pu convert P"/1 -> "mQ droop "/1
  Transfer Fcn1/1 -> " pu convert S"/1
  " pu convert S"/1 -> limiter/1(In1), Sum2/2
  i_meas/1 -> 3-phase  Instantaneous  Active & Reactive Power/2
  P_req/1 -> Sum2/1
  mP droop/1 -> Sum3/2
  limiter/1(Out1) -> Sum3/1, k/1
  w0/1 -> Sum3/3
  Sum2/1 -> mP droop/1
  Sum1/1 -> PI-Control/1(In1)
  Sum/1 -> Sum1/1
  "mQ droop "/1 -> Sum/1
  RMS/1 -> Transfer Fcn2/1
  Demux/2 -> Transfer Fcn/1
  Demux/1 -> Transfer Fcn1/1
  3-phase  Instantaneous  Active & Reactive Power/1 -> Demux/1
  v_meas/1 -> RMS/1, 3-phase  Instantaneous  Active & Reactive Power/1
  PI-Control/1(Out1) -> Vpk/1
  Sum3/1 -> w/1
  E_req/1 -> Sum/2
  " pu convert V"/1 -> Sum1/2
  k/1 -> Pmm/1

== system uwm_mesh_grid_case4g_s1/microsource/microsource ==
  Vpk : Inport  OutDataType=fixdt(1, 16)  OutScaling=2^0
  w : Inport  Port=2  OutDataType=fixdt(1, 16)  OutScaling=2^0
  Demux : Demux  Outputs=3
  Ground2 : powerlib/Elements/Ground  DialogController=POWERSYS.PowerSysDialog  PhysicalDomain=powersysdomain  SubClassName=unknown  LeftPortType=p1  RightPortType=p1  LConnTagsString=a
  Integrator : Integrator
  Mux : Mux  Inputs=3
  Product : Product  OutDataType=sfix(16)  OutScaling=2^0
  Series RLC Branch : powerlib/Elements/Series RLC Branch  DialogController=POWERSYS.PowerSysDialog  PhysicalDomain=powersysdomain  SubClassName=unknown  LeftPortType=p1  RightPortType=p1  LConnTagsString=__new0  RConnTagsString=__new0  BranchType=C  Resistance=1  Inductance=1e-3  SetiL0=off  InitialCurrent=0  Capacitance=1e-8  Setx0=off  InitialVoltage=0  Measurements=None
  phaseA : powerlib/Electrical Sources/Controlled Voltage Source  DialogController=POWERSYS.PowerSysDialog  SystemSampleTime=-1  Initialize=on  Source_Type=AC  Amplitude=0  Phase=0  Frequency=0  Measurements=None
  phaseB : powerlib/Electrical Sources/Controlled Voltage Source  DialogController=POWERSYS.PowerSysDialog  SystemSampleTime=-1  Initialize=on  Source_Type=AC  Amplitude=0  Phase=0  Frequency=0  Measurements=None
  phaseC : powerlib/Electrical Sources/Controlled Voltage Source  DialogController=POWERSYS.PowerSysDialog  SystemSampleTime=-1  Initialize=on  Source_Type=AC  Amplitude=0  Phase=0  Frequency=0  Measurements=None
  v_A : Fcn  Expr=cos(u)
  v_B : Fcn  Expr=cos(u-2*pi/3)
  v_C : Fcn  Expr=cos(u+2*pi/3)
  Va : PMIOPort  Tag=PMCPort  Port=1  Side=Right
  Vb : PMIOPort  Tag=PMCPort  Port=2  Side=Right
  Vc : PMIOPort  Tag=PMCPort  Port=3  Side=Right
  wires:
  Product/1 -> Demux/1
  Vpk/1 -> Product/1
  Mux/1 -> Product/2
  w/1 -> Integrator/1
  Integrator/1 -> v_A/1, v_B/1, v_C/1
  v_A/1 -> Mux/1
  v_B/1 -> Mux/2
  v_C/1 -> Mux/3
  Demux/1 -> phaseA/1
  Demux/2 -> phaseB/1
  Demux/3 -> phaseC/1
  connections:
  Vb/RConn1 -- phaseB/RConn1 -- phaseA/LConn1
  Va/RConn1 -- phaseC/LConn1 -- phaseA/RConn1
  Vc/RConn1 -- phaseC/RConn1
  Series RLC Branch/RConn1 -- Ground2/LConn1
  Series RLC Branch/LConn1 -- phaseB/LConn1

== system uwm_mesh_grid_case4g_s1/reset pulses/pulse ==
  Step : Step  Time=tstart  SampleTime=0
  Step1 : Step  Time=tstart+dt  After=-1  SampleTime=0
  Sum : Sum  Inputs=|++  OutDataType=fixdt(1, 16)  OutScaling=2^0
  Out1 : Outport
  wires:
  Step/1 -> Sum/2
  Step1/1 -> Sum/1
  Sum/1 -> Out1/1

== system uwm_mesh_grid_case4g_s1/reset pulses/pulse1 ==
  Step : Step  Time=tstart  SampleTime=0
  Step1 : Step  Time=tstart+dt  After=-1  SampleTime=0
  Sum : Sum  Inputs=|++  OutDataType=fixdt(1, 16)  OutScaling=2^0
  Out1 : Outport
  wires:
  Step/1 -> Sum/2
  Step1/1 -> Sum/1
  Sum/1 -> Out1/1

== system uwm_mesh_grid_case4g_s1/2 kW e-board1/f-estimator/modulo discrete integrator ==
  In1 : Inport
  Abs : Abs
  Constant1 : Constant  OutDataType=sfix(16)  OutScaling=2^0
  Discrete-Time Integrator : DiscreteIntegrator  ExternalReset=rising  InitialConditionSource=external  SampleTime=dt  OutDataType=fixdt(1, 16)  OutScaling=2^0  UpperSaturationLimit=100  LowerSaturationLimit=-100  ShowStatePort=on  ICPrevOutput=DiscIntNeverNeededParam  ICPrevScaledInput=DiscIntNeverNeededParam
  Gain1 : Gain  Gain=1+.0001  ParameterDataType=sfix(16)  ParameterScaling=2^0  OutDataType=sfix(16)  OutScaling=2^0
  IC : InitialCondition  Value=0
  Math Function : Math  Operator=rem  OutDataType=sfix(16)  OutScaling=2^0
  Relational Operator : RelationalOperator
  Out1 : Outport
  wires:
  Math Function/1 -> IC/1
  IC/1 -> Discrete-Time Integrator/3
  Discrete-Time Integrator/1 -> Out1/1
  In1/1 -> Discrete-Time Integrator/1
  Abs/1 -> Math Function/1, Relational Operator/1
  Constant1/1 -> Math Function/2, Relational Operator/2
  Gain1/1 -> Abs/1
  Discrete-Time Integrator/State -> Gain1/1
  Relational Operator/1 -> Discrete-Time Integrator/2

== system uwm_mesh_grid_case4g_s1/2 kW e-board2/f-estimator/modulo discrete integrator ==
  In1 : Inport
  Abs : Abs
  Constant1 : Constant  OutDataType=sfix(16)  OutScaling=2^0
  Discrete-Time Integrator : DiscreteIntegrator  ExternalReset=rising  InitialConditionSource=external  SampleTime=dt  OutDataType=fixdt(1, 16)  OutScaling=2^0  UpperSaturationLimit=100  LowerSaturationLimit=-100  ShowStatePort=on  ICPrevOutput=DiscIntNeverNeededParam  ICPrevScaledInput=DiscIntNeverNeededParam
  Gain1 : Gain  Gain=1+.0001  ParameterDataType=sfix(16)  ParameterScaling=2^0  OutDataType=sfix(16)  OutScaling=2^0
  IC : InitialCondition  Value=0
  Math Function : Math  Operator=rem  OutDataType=sfix(16)  OutScaling=2^0
  Relational Operator : RelationalOperator
  Out1 : Outport
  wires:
  Math Function/1 -> IC/1
  IC/1 -> Discrete-Time Integrator/3
  Discrete-Time Integrator/1 -> Out1/1
  In1/1 -> Discrete-Time Integrator/1
  Abs/1 -> Math Function/1, Relational Operator/1
  Constant1/1 -> Math Function/2, Relational Operator/2
  Gain1/1 -> Abs/1
  Discrete-Time Integrator/State -> Gain1/1
  Relational Operator/1 -> Discrete-Time Integrator/2

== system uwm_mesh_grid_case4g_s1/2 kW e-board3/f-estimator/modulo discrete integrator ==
  In1 : Inport
  Abs : Abs
  Constant1 : Constant  OutDataType=sfix(16)  OutScaling=2^0
  Discrete-Time Integrator : DiscreteIntegrator  ExternalReset=rising  InitialConditionSource=external  SampleTime=dt  OutDataType=fixdt(1, 16)  OutScaling=2^0  UpperSaturationLimit=100  LowerSaturationLimit=-100  ShowStatePort=on  ICPrevOutput=DiscIntNeverNeededParam  ICPrevScaledInput=DiscIntNeverNeededParam
  Gain1 : Gain  Gain=1+.0001  ParameterDataType=sfix(16)  ParameterScaling=2^0  OutDataType=sfix(16)  OutScaling=2^0
  IC : InitialCondition  Value=0
  Math Function : Math  Operator=rem  OutDataType=sfix(16)  OutScaling=2^0
  Relational Operator : RelationalOperator
  Out1 : Outport
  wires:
  Math Function/1 -> IC/1
  IC/1 -> Discrete-Time Integrator/3
  Discrete-Time Integrator/1 -> Out1/1
  In1/1 -> Discrete-Time Integrator/1
  Abs/1 -> Math Function/1, Relational Operator/1
  Constant1/1 -> Math Function/2, Relational Operator/2
  Gain1/1 -> Abs/1
  Discrete-Time Integrator/State -> Gain1/1
  Relational Operator/1 -> Discrete-Time Integrator/2
